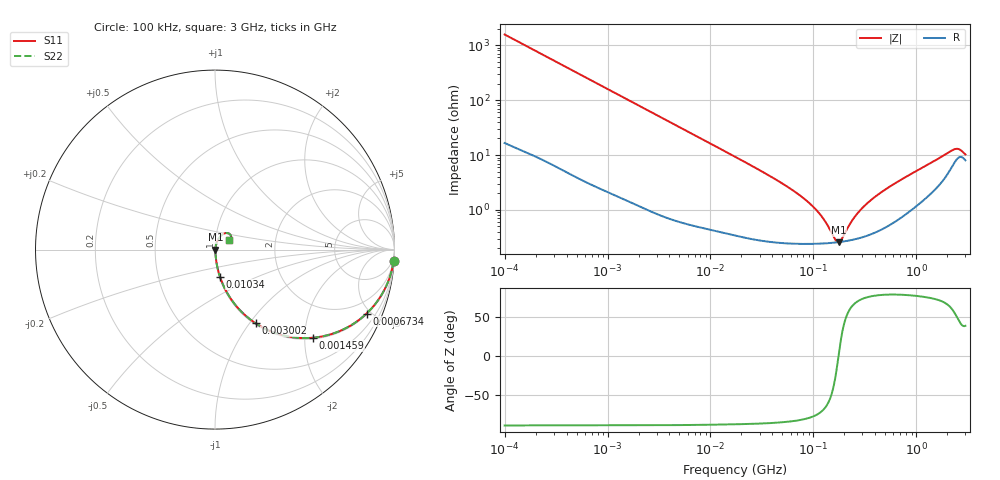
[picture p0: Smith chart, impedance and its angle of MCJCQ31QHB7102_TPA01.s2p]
! MCJCQ31QHB7102_TPA01  S-PARAMETER MODEL  ( Standard Model )
! Model Generated by TAIYO YUDEN Corporation (http://www.ty-top.com)
! Version 1.0
! TAIYO YUDEN Control No. 220601
! Copyright(c) 2015 TAIYO YUDEN CO.,LTD. All Rights Reserved.
! Product Description (link to TY-COMPAS)
! https://ds.yuden.co.jp/TYCOMPAS/or/detail?pn=MCJCQ31QHB7102KTPA01&u=M
! Products Name : Multilayer Ceramic Capacitors
! Characteristics :
!  Capacitance : 1000 [pF] , Rated Voltage : 250 [V] , TCC : X7R
!  Case Size : 3.2 x 1.6 / 0.126 x 0.063 [mm/inch] , Thickness : 1.15 / 0.045 [mm/inch]
!  (Conditions: Temperature = 25 [degC] , DC Bias Voltage = 0 [V])
! External Node Assignments :
!  1  o---| |---o  2
! GND o---------o GND
! Frequency Range : 100kHz  -  3GHz  [ 401 STEP ]
# MHZ S RI R 50
! Freq[MHz].  S11 Real  S11 Imag  S21 Real  S21 Imag  S12 Real  S12 Imag  S22 Real  S22 Imag
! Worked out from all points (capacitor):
!   401 points, 100 kHz to 3 GHz, reference 50 ohm
!   read as one part in series: C = 1.02 nF near 105.3 kHz
!   lowest |Z| = 259 mohm at 176.2 MHz (marker M1)
!   series resonance near 175.7 MHz, so ESL is about 810 pH
!   S11 on the Smith chart (normalised r, x): 100 kHz: 1, -31; 673.4 kHz: 1.06, -4.71; 1.459 MHz: 1.03, -2.19; 3.002 MHz: 1.02, -1.07; 10.34 MHz: 1.01, -0.31; 3 GHz: 1.16, +0.13
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0.1  0.9953 -0.0636  0.00474 0.0636  0.00474 0.0636  0.9953 -0.0636
0.246461  0.9743 -0.1523  0.0257 0.1523  0.0257 0.1523  0.9743 -0.1523
0.562235  0.8851 -0.3128  0.1149 0.3128  0.1149 0.3128  0.8851 -0.3128
0.673391  0.8441 -0.3565  0.1559 0.3565  0.1559 0.3565  0.8441 -0.3565
1.458987  0.5439 -0.491  0.4561 0.491  0.4561 0.491  0.5439 -0.491
3.002272  0.2257 -0.4102  0.7743 0.4102  0.7743 0.4102  0.2257 -0.4102
3.161081  0.2086 -0.3984  0.7914 0.3984  0.7914 0.3984  0.2086 -0.3984
5.292876  0.089 -0.2753  0.911 0.2753  0.911 0.2753  0.089 -0.2753
10.34438  0.0277 -0.151  0.9723 0.151  0.9723 0.151  0.0277 -0.151
17.7727  0.0115 -0.0894  0.9885 0.0894  0.9885 0.0894  0.0115 -0.0894
53.83243  0.00322 -0.0275  0.9968 0.0275  0.9968 0.0275  0.00322 -0.0275
97.38194  0.00254 -0.0116  0.9975 0.0116  0.9975 0.0116  0.00254 -0.0116
126.0104  0.00249 -0.00629  0.9975 0.00629  0.9975 0.00629  0.00249 -0.00629
163.0551  0.00255 -0.00139  0.9975 0.00139  0.9975 0.00139  0.00255 -0.00139
176.1623  0.00259 5.2e-05  0.9974 -5.2e-05  0.9974 -5.2e-05  0.00259 5.2e-05
190.323  0.00264 0.00149  0.9974 -0.00149  0.9974 -0.00149  0.00264 0.00149
233.9019  0.00285 0.00538  0.9971 -0.00538  0.9971 -0.00538  0.00285 0.00538
287.4592  0.00319 0.00949  0.9968 -0.00949  0.9968 -0.00949  0.00319 0.00949
547.5153  0.00588 0.0255  0.9941 -0.0255  0.9941 -0.0255  0.00588 0.0255
2201.951  0.0651 0.0925  0.9349 -0.0925  0.9349 -0.0925  0.0651 0.0925
2570.185  0.0886 0.0773  0.9114 -0.0773  0.9114 -0.0773  0.0886 0.0773
3000  0.0773 0.0543  0.9227 -0.0543  0.9227 -0.0543  0.0773 0.0543
